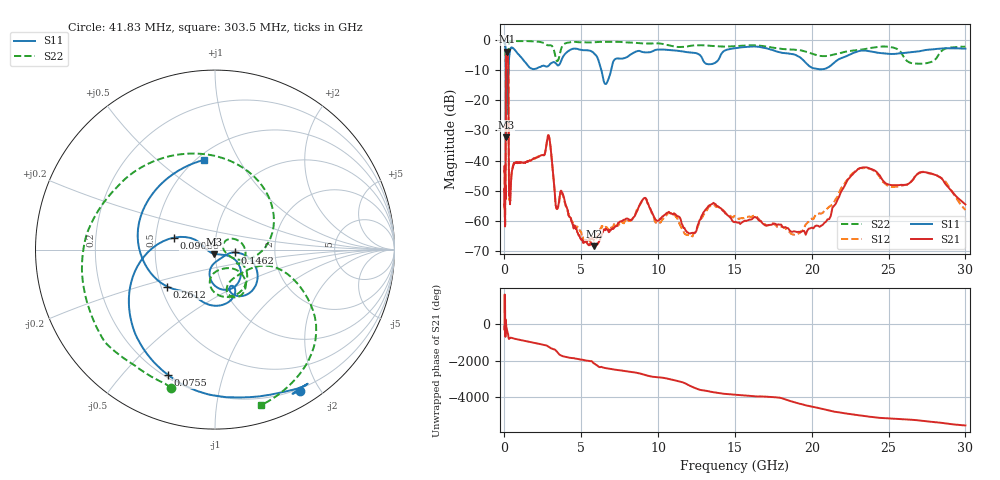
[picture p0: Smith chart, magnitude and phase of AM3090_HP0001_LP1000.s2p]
! Date/Time: Thu, Feb 28, 2019 1:54 PM
! Network Analyzer: Agilent Technologies E8364B Rev: A.07.50.67
! Sweep from 0.010 to 30.000 GHz, 1601 Points, Sweep Type: LOG
! Power Supply: 5.023 V, 0.002 A
# Hz S DB R 50
!freq MagS11 AngS11 MagS21 AngS21 MagS12 AngS12 MagS22 AngS22
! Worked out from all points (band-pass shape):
!   1601 points, 10 MHz to 30 GHz, reference 50 ohm
!   highest |S21| = -3.84 dB at 147.6 MHz (marker M1); lowest = -68.4 dB at 5.812 GHz (marker M2)
!   |S21| within 3 dB of the highest: 99.96 MHz to 238.5 MHz (138.6 MHz wide, 81.9 % of centre)
!   lowest |S11| = -32.3 dB at 98.93 MHz (marker M3), VSWR 1.05, Z = 49.5 - j2.36 ohm
!   |S11| at or under -10 dB: 89.58 MHz to 258.1 MHz (168.5 MHz wide, 96.9 % of centre); 6.308 GHz to 6.937 GHz (629 MHz wide, 9.5 % of centre)
!   |S22| runs from -26.7 to -0.1 dB; largest |S21 - S12| = 0.014
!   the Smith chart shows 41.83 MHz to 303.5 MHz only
!   S11 on the Smith chart (normalised r, x): 41.83 MHz: 0.17, -1.75; 75.5 MHz: 0.21, -0.67; 90.86 MHz: 0.63, +0.09; 146.2 MHz: 1.25, -0.04; 261.2 MHz: 0.54, -0.25; 303.5 MHz: 0.54, +0.73
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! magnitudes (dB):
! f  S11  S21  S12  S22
! 10 MHz  -0.2  -43.6  -44.2  -0.6
! 38.04 MHz  -0.5  -60.5  -59.0  -1.5
! 41.83 MHz  -0.7  -60.7  -60.8  -1.9
! 75.5 MHz  -2.5  -45.9  -43.8  -4.7
! 90.86 MHz  -12.5  -14.2  -14.2  -11.6
! 98.93 MHz  -32.3  -7.2  -7.2  -25.8
! 115 MHz  -12.8  -4.9  -4.9  -17.3
! 144.7 MHz  -20.6  -3.9  -3.8  -16.5
! 146.2 MHz  -18.9  -3.8  -3.8  -16.3
! 147.6 MHz  -17.4  -3.8  -3.8  -15.9
! 261.2 MHz  -9.5  -15.2  -15.1  -9.7
! 303.5 MHz  -6.0  -50.5  -51.2  -0.9
! 550.5 MHz  -2.7  -42.0  -41.8  -0.2
! 2.084 GHz  -9.5  -39.0  -38.9  -0.5
! 2.884 GHz  -8.5  -31.7  -31.8  -1.7
! 3.402 GHz  -8.1  -56.0  -56.0  -6.9
! 5.812 GHz  -4.3  -68.4  -66.5  -0.7
! 6.619 GHz  -14.5  -62.9  -62.1  -0.6
! 7.926 GHz  -5.8  -59.2  -60.5  -0.8
! 19.31 GHz  -6.0  -63.7  -63.4  -3.4
! 23.36 GHz  -3.5  -42.2  -42.5  -3.1
! 30 GHz  -2.9  -54.5  -56.4  -2.2
